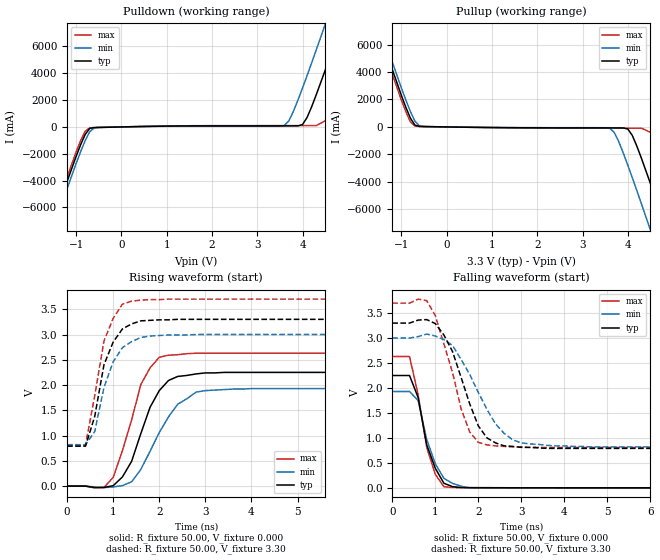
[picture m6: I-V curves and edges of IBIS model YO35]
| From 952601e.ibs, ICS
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|   Model YO35
[Model]   YO35
Model_type   Output
Polarity   Non-Inverting
C_comp   5.50pF   5.00pF   6.00pF
[Temperature Range]   27.00   70.00   0.000
[Voltage Range]   3.30V   3.00V   3.70V
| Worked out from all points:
|   slope of the pulldown table from 0 to 0.495 V, typ, clamps not added: 14.3 ohm
|   slope of the pullup table from 0 to 0.495 V, typ, clamps not added: 20.5 ohm
|   rising waveform, R_fixture 50.00, V_fixture 0.000: 20-80 % time 571ps typ, 708ps min, 523ps max; typ from 0 V to 2.25 V
|   rising waveform, R_fixture 50.00, V_fixture 3.30: 20-80 % time 407ps typ, 434ps min, 394ps max; typ from 0.79 V to 3.3 V
|   falling waveform, R_fixture 50.00, V_fixture 0.000: 20-80 % time 372ps typ, 412ps min, 367ps max; typ from 2.25 V to 0 V
|   falling waveform, R_fixture 50.00, V_fixture 3.30: 20-80 % time 620ps typ, 821ps min, 568ps max; typ from 3.3 V to 0.78 V
[Pulldown]
| voltage   I(typ)   I(min)   I(max)
-3.3V     -24.56A    -25.23A    -24.25A
-1.7V     -8.83A     -9.35A     -8.5A
-1.5V     -6.89A     -7.42A     -6.56A
-900mV    -1.32A     -1.84A     -1.01A
-700mV    -110mA     -360mA     -66.3mA
3.6V      78.43mA    110mA      96.66mA
4V        180mA      2.91A      96.96mA
4.3V      2.38A      5.72A      97.64mA
4.5V      4.23A      7.64A      450mA
4.9V      8.07A      11.53A     3.91A
5.3V      11.98A     15.45A     7.76A
6.6V      24.84A     28.32A     20.57A
[Pullup]
| voltage   I(typ)   I(min)   I(max)
-3.3V     24.68A     25.19A     24.36A
-1.7V     8.94A      9.48A      8.6A
-1.5V     7.01A      7.55A      6.66A
-900mV    1.42A      1.95A      1.1A
-700mV    130mA      420mA      59.96mA
3.6V      -71.58mA   -89.94mA   -90.05mA
4V        -150mA     -2.79A     -91.24mA
4.3V      -2.27A     -5.59A     -92.46mA
4.5V      -4.12A     -7.51A     -390mA
4.9V      -7.96A     -11.4A     -3.8A
5.3V      -11.88A    -15.32A    -7.65A
6.6V      -24.75A    -28.2A     -20.48A
[Ramp]
| variable   typ   min   max
dV/dt_r   1.35/0.55n   1.16/0.69n   1.58/0.43n
dV/dt_f   1.51/0.60n   1.31/0.81n   1.74/0.48n
R_load = 50.00
[Rising Waveform]
R_fixture = 50.00
V_fixture = 0.000
V_fixture_min = 0.000
V_fixture_max = 0.000
| time   V(typ)   V(min)   V(max)
0s        190uV      61.32uV    270uV
800ps     -26.94mV   -28.9mV    -25.4mV
1ns       8.07mV     -16.13mV   170mV
1.4ns     490mV      86.35mV    1.31V
1.6ns     1.04V      330mV      2.01V
1.8ns     1.56V      690mV      2.34V
2ns       1.89V      1.06V      2.55V
2.4ns     2.17V      1.62V      2.6V
3ns       2.24V      1.89V      2.63V
10ns      2.25V      1.93V      2.63V
[Rising Waveform]
R_fixture = 50.00
V_fixture = 3.30
V_fixture_min = 3.00
V_fixture_max = 3.70
| time   V(typ)   V(min)   V(max)
0s        790mV      820mV      810mV
400ps     790mV      820mV      810mV
600ps     1.38V      1.08V      1.79V
800ps     2.4V       1.95V      2.87V
1ns       2.85V      2.46V      3.32V
1.2ns     3.11V      2.74V      3.6V
1.4ns     3.21V      2.86V      3.66V
1.8ns     3.28V      2.97V      3.69V
2.8ns     3.3V       3V         3.7V
10ns      3.3V       3V         3.7V
[Falling Waveform]
R_fixture = 50.00
V_fixture = 0.000
V_fixture_min = 0.000
V_fixture_max = 0.000
| time   V(typ)   V(min)   V(max)
0s        2.25V      1.93V      2.63V
400ps     2.25V      1.93V      2.63V
600ps     1.81V      1.75V      1.87V
800ps     860mV      970mV      810mV
1ns       390mV      480mV      270mV
1.2ns     90.98mV    190mV      22.17mV
1.4ns     23.83mV    88.57mV    6.54mV
1.6ns     5.19mV     32.24mV    3.54mV
1.8ns     3.2mV      -830uV     2.71mV
10ns      -2.36uV    -29.17uV   -5.11uV
[Falling Waveform]
R_fixture = 50.00
V_fixture = 3.30
V_fixture_min = 3.00
V_fixture_max = 3.70
| time   V(typ)   V(min)   V(max)
0s        3.3V       3V         3.7V
800ps     3.37V      3.08V      3.75V
1ns       3.29V      3.04V      3.45V
1.4ns     2.73V      2.85V      2.31V
1.6ns     2.21V      2.57V      1.58V
1.8ns     1.68V      2.27V      1.12V
2ns       1.24V      1.91V      910mV
2.4ns     900mV      1.28V      840mV
3ns       810mV      900mV      820mV
10ns      780mV      820mV      810mV
